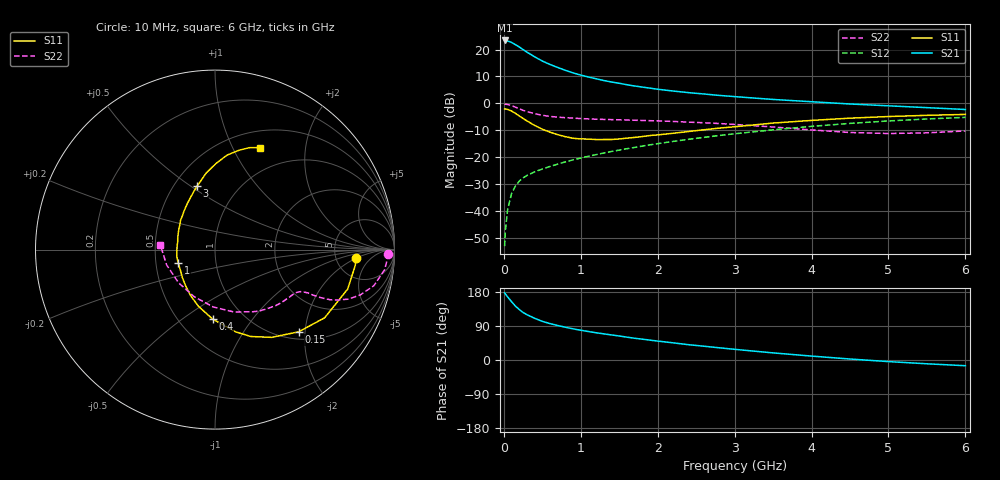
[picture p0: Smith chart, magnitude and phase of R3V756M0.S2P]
! SIEMENS Small Signal Semiconductors
! BFR181
! Si NPN RF Bipolar Junction Transistor in SOT23
! VCE = 0.75 V  IC = 6 mA
! Common Emitter S-Parameters:  May  1996
# GHz  S  MA  R  50
!  f  S11  S21  S12  S22
! GHz  MAG  ANG  MAG  ANG  MAG  ANG  MAG  ANG
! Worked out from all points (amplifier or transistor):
!   36 points, 10 MHz to 6 GHz, reference 50 ohm
!   highest |S21| = 23.4 dB at 10 MHz (marker M1)
!   |S21| within 3 dB of that: start of sweep to 229.6 MHz
!   unconditionally stable (mu >= 1): 655 MHz to 3.629 GHz
!   at 250 MHz: K = 0.56, MSG = 23.9 dB, |S12| = -27.7 dB
!   at 1.4 GHz: K = 1.19, MAG = 10.3 dB, |S12| = -17.9 dB
!   at 6 GHz: K = 0.96, MSG = 1.5 dB, |S12| = -5.2 dB
!   S11 on the Smith chart (normalised r, x): 10 MHz: 7.85, -1.97; 150 MHz: 1.16, -1.85; 400 MHz: 0.72, -0.66; 1 GHz: 0.65, -0.10; 3 GHz: 0.65, +0.53; 6 GHz: 0.69, +1.29
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0.01  0.7862 -3.5  14.8 177.3  0.0022 88.2  0.9665 -1.3
0.02  0.7866 -6.4  14.58 174.4  0.0043 87.7  0.9626 -2.8
0.05  0.7711 -16.6  14.47 166.4  0.0108 81.4  0.9516 -6.8
0.1  0.7192 -31.9  13.64 153.9  0.0209 74.2  0.9077 -12.8
0.15  0.6534 -44.5  12.38 142.4  0.0288 68.0  0.8495 -17.2
0.2  0.5823 -57.1  11.2 133.3  0.0357 65.1  0.7945 -20.3
0.25  0.5237 -67.6  10.01 125.4  0.041 61.6  0.741 -22.3
0.3  0.4714 -76.1  8.981 119.6  0.0455 60.5  0.702 -23.5
0.4  0.3883 -91.8  7.364 110.1  0.0531 59.3  0.6431 -24.5
0.5  0.3298 -106.0  6.127 102.0  0.0599 59.3  0.6 -24.9
0.6  0.291 -117.6  5.288 96.1  0.067 59.9  0.5713 -25.0
0.8  0.2398 -139.3  4.121 86.5  0.0815 60.8  0.5412 -25.7
1  0.218 -160.1  3.357 78.5  0.0961 62.1  0.5213 -26.9
1.1  0.2163 -170.0  3.094 75.1  0.1036 62.6  0.5136 -27.7
1.3  0.2122 175.0  2.659 68.9  0.1193 62.9  0.5025 -29.6
1.6  0.2252 155.2  2.222 60.3  0.1433 62.4  0.4901 -33.2
2.2  0.2773 128.1  1.697 45.3  0.1956 60.2  0.4609 -42.5
3  0.3665 105.9  1.335 28.2  0.2713 54.4  0.4053 -58.7
3.5  0.4299 96.5  1.182 18.7  0.322 49.6  0.3632 -73.1
4.5  0.5303 82.8  0.973 2.6  0.4237 37.4  0.2868 -113.9
5.5  0.5987 71.5  0.832 -10.0  0.5119 23.8  0.2827 -162.4
6  0.6226 66.0  0.769 -15.1  0.5491 16.4  0.3064 174.9
